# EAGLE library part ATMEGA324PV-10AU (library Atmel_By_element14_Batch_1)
8-bit Microcontroller with 16K/32K/64K Bytes In-System Programmable Flash
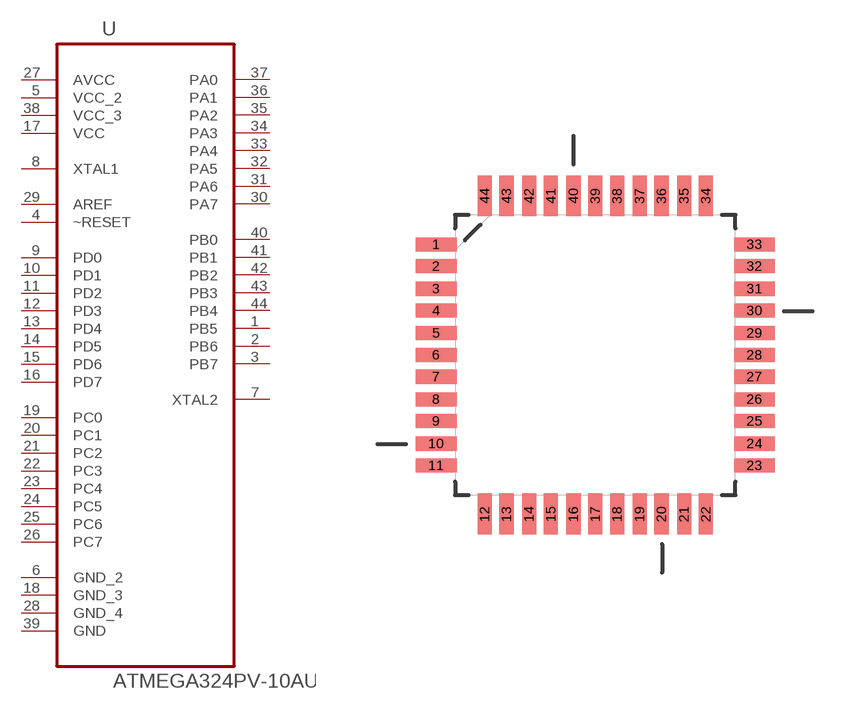
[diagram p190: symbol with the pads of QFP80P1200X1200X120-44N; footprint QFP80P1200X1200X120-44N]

Designator prefix U

## ATMEGA324PV-10AU (MPN: ATMEGA324PV-10AU; OC_FARNELL: 1455111; OC_NEWARK: 58M3737; PACKAGE: TQFP-44; SUPPLIER: Atmel)  [QFP80P1200X1200X120-44N]
1  PB5
2  PB6
3  PB7
4  ~RESET  in
5  VCC_2  pwr
6  GND_2  pas
7  XTAL2  out
8  XTAL1  in
9  PD0
10  PD1
11  PD2
12  PD3
13  PD4
14  PD5
15  PD6
16  PD7
17  VCC  pwr
18  GND_3  pas
19  PC0
20  PC1
21  PC2
22  PC3
23  PC4
24  PC5
25  PC6
26  PC7
27  AVCC  pwr
28  GND_4  pas
29  AREF  in
30  PA7
31  PA6
32  PA5
33  PA4
34  PA3
35  PA2
36  PA1
37  PA0
38  VCC_3  pwr
39  GND  pas
40  PB0
41  PB1
42  PB2
43  PB3
44  PB4

## Footprint QFP80P1200X1200X120-44N (pad centres in mm)
smd 1.473 x 0.508: 1 -5.74,3.988; 2 -5.74,3.2; 3 -5.74,2.388; 4 -5.74,1.6; 5 -5.74,0.787; 6 -5.74,0; 7 -5.74,-0.787; 8 -5.74,-1.6; 9 -5.74,-2.388; 10 -5.74,-3.2; 11 -5.74,-3.988; 23 5.74,-3.988; 24 5.74,-3.2; 25 5.74,-2.388; 26 5.74,-1.6; 27 5.74,-0.787; 28 5.74,0; 29 5.74,0.787; 30 5.74,1.6; 31 5.74,2.388; 32 5.74,3.2; 33 5.74,3.988
smd 0.508 x 1.473: 12 -3.988,-5.74; 13 -3.2,-5.74; 14 -2.388,-5.74; 15 -1.6,-5.74; 16 -0.787,-5.74; 17 0,-5.74; 18 0.787,-5.74; 19 1.6,-5.74; 20 2.388,-5.74; 21 3.2,-5.74; 22 3.988,-5.74; 34 3.988,5.74; 35 3.2,5.74; 36 2.388,5.74; 37 1.6,5.74; 38 0.787,5.74; 39 0,5.74; 40 -0.787,5.74; 41 -1.6,5.74; 42 -2.388,5.74; 43 -3.2,5.74; 44 -3.988,5.74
